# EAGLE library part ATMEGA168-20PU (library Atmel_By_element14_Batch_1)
Microcontroller
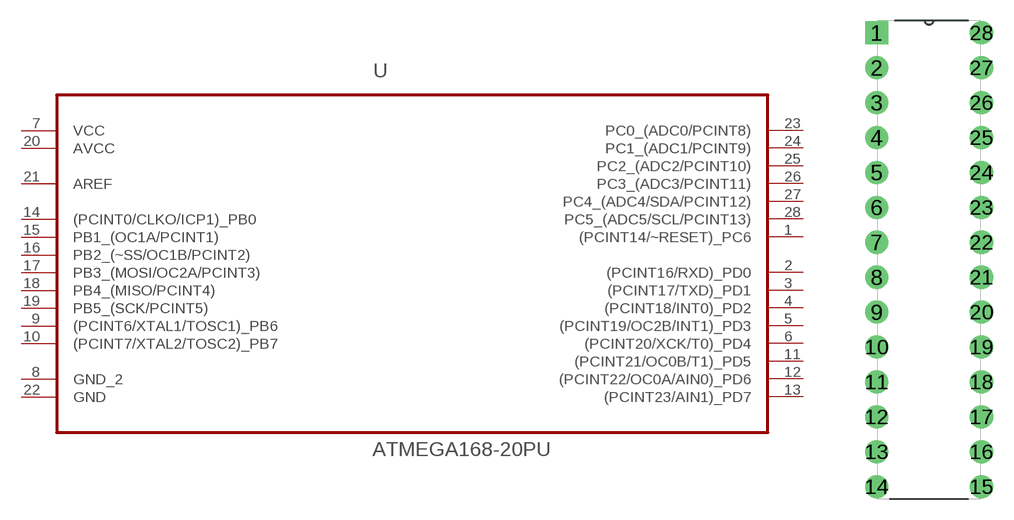
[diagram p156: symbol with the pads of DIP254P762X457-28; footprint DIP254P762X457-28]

Designator prefix U

## ATMEGA168-20PU (DESCRIPTION: Microcontroller; MPN: ATMEGA168-20PU; OC_FARNELL: 9171207; OC_NEWARK: 01M6892; PACKAGE: PCDIP-28; SUPPLIER: ATMEL)  [DIP254P762X457-28]
1  (PCINT14/~RESET)_PC6
2  (PCINT16/RXD)_PD0
3  (PCINT17/TXD)_PD1
4  (PCINT18/INT0)_PD2
5  (PCINT19/OC2B/INT1)_PD3
6  (PCINT20/XCK/T0)_PD4
7  VCC  pwr
8  GND_2  pas
9  (PCINT6/XTAL1/TOSC1)_PB6
10  (PCINT7/XTAL2/TOSC2)_PB7
11  (PCINT21/OC0B/T1)_PD5
12  (PCINT22/OC0A/AIN0)_PD6
13  (PCINT23/AIN1)_PD7
14  (PCINT0/CLKO/ICP1)_PB0
15  PB1_(OC1A/PCINT1)
16  PB2_(~SS/OC1B/PCINT2)
17  PB3_(MOSI/OC2A/PCINT3)
18  PB4_(MISO/PCINT4)
19  PB5_(SCK/PCINT5)
20  AVCC  pwr
21  AREF  in
22  GND  pas
23  PC0_(ADC0/PCINT8)
24  PC1_(ADC1/PCINT9)
25  PC2_(ADC2/PCINT10)
26  PC3_(ADC3/PCINT11)
27  PC4_(ADC4/SDA/PCINT12)
28  PC5_(ADC5/SCL/PCINT13)

## Footprint DIP254P762X457-28 (pad centres in mm)
drill 1.118 square: 1 -7.62,33.02
drill 1.118: 2 -7.62,30.48; 3 -7.62,27.94; 4 -7.62,25.4; 5 -7.62,22.86; 6 -7.62,20.32; 7 -7.62,17.78; 8 -7.62,15.24; 9 -7.62,12.7; 10 -7.62,10.16; 11 -7.62,7.62; 12 -7.62,5.08; 13 -7.62,2.54; 14 -7.62,0; 15 0,0; 16 0,2.54; 17 0,5.08; 18 0,7.62; 19 0,10.16; 20 0,12.7; 21 0,15.24; 22 0,17.78; 23 0,20.32; 24 0,22.86; 25 0,25.4; 26 0,27.94; 27 0,30.48; 28 0,33.02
